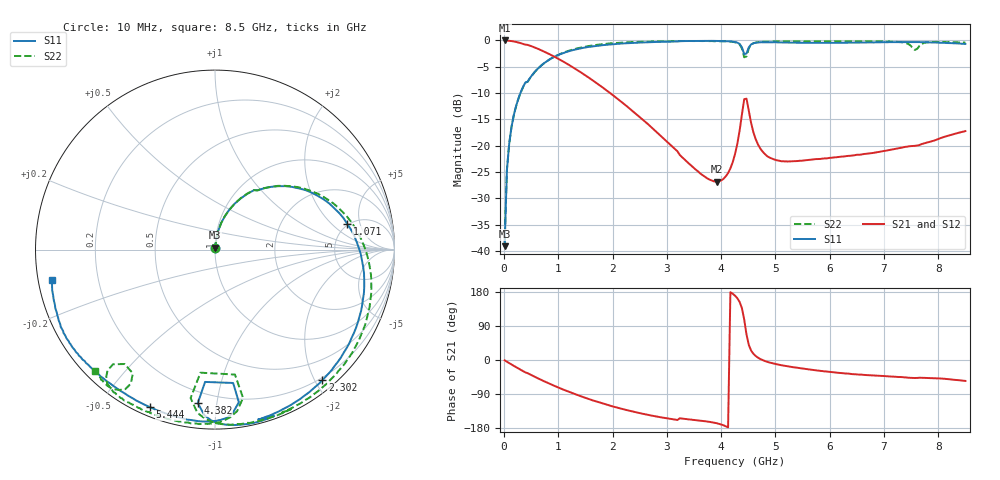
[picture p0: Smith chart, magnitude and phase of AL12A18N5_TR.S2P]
!AVX CORPORATION
!PART NUMBER AL12A18N5_TR
!DESCRIPTION: AIR CORE INDUCTOR, 18.5nH, 5 TURNS
!Agilent Technologies,E5071C,MY46102230,A.09.54
!Date: Mon Sep 03 15:46:28 2012
!Data & Calibration Information:
!Freq	S11:SOLT2(ON)	S21:SOLT2(ON)	S12:SOLT2(ON)	S22:SOLT2(ON)
# Hz S RI R 50
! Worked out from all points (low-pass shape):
!   201 points, 10 MHz to 8.5 GHz, reference 50 ohm
!   highest |S21| = -0.02 dB at 10 MHz (marker M1); lowest = -26.8 dB at 3.915 GHz (marker M2)
!   |S21| within 3 dB of the highest: start of sweep to 911.3 MHz
!   lowest |S11| = -39.1 dB at 10 MHz (marker M3), VSWR 1.02, Z = 50.1 + j1.1 ohm
!   |S11| at or under -10 dB: start of sweep to 302 MHz
!   |S22| runs from -38.9 to -0.1 dB; largest |S21 - S12| = 0.012
!   S11 on the Smith chart (normalised r, x): 10 MHz: 1.00, +0.02; 1.071 GHz: 4.88, +3.19; 2.302 GHz: 0.16, -2.10; 4.382 GHz: 0.13, -0.88; 5.444 GHz: 0.04, -0.67; 8.5 GHz: 0.04, -0.09
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1e7  0.0015 0.011  0.9979 -0.0153  1.006 -0.024  0.00117 0.0113
5.245e7  0.00679 0.0581  0.9924 -0.0797  0.9969 -0.0818  0.00687 0.0586
1.3735e8  0.0335 0.1469  0.9635 -0.2024  0.9655 -0.2033  0.0342 0.1466
2.2225e8  0.0812 0.2246  0.9137 -0.3143  0.9147 -0.3153  0.0815 0.2231
6.043e8  0.392 0.3536  0.5726 -0.6141  0.5728 -0.6156  0.3872 0.3555
1.07125e9  0.7372 0.1425  0.1445 -0.6206  0.1439 -0.6211  0.734 0.1854
1.4533e9  0.8313 -0.1685  -0.0646 -0.4776  -0.0649 -0.4775  0.8588 -0.0784
2.3023e9  0.5973 -0.7282  -0.157 -0.1645  -0.1571 -0.1644  0.7362 -0.6155
2.85415e9  0.37 -0.8945  -0.1117 -0.0637  -0.1118 -0.0634  0.5191 -0.8291
3.9154e9  0.1614 -0.9736  -0.0444 -0.0105  -0.0442 -0.0104  0.1597 -0.9693
4.255e9  0.0104 -0.9642  -0.0817 0.0147  -0.0816 0.0149  -0.0185 -0.9586
4.38235e9  -0.096 -0.855  -0.1442 0.135  -0.1442 0.1352  -0.1358 -0.827
4.4248e9  -0.0553 -0.7373  -0.0798 0.2648  -0.0795 0.2649  -0.0809 -0.6857
4.5097e9  0.1329 -0.8501  0.1642 0.1361  0.1642 0.1359  0.1564 -0.8264
4.80685e9  -0.0712 -0.9575  0.0829 -0.00405  0.083 -0.00406  -0.0394 -0.9713
5.4436e9  -0.3613 -0.878  0.0668 -0.0262  0.0668 -0.0263  -0.2475 -0.9465
5.6983e9  -0.4561 -0.8299  0.0662 -0.0329  0.0659 -0.0329  -0.3134 -0.9256
7.09915e9  -0.7722 -0.5737  0.066 -0.0624  0.0661 -0.0624  -0.5652 -0.7949
7.4812e9  -0.8218 -0.5016  0.0673 -0.0723  0.0676 -0.0727  -0.5984 -0.6731
7.60855e9  -0.8383 -0.4725  0.0678 -0.0736  0.0677 -0.0733  -0.4579 -0.6894
7.7359e9  -0.8532 -0.4409  0.0713 -0.0769  0.0711 -0.077  -0.5306 -0.7819
8.5e9  -0.9094 -0.1693  0.0785 -0.1128  0.0789 -0.1128  -0.6689 -0.6772
